PROGRAM p10_directionalInterlock
VAR
	interlockS0: TOF;
	interlockS1: TOF;
	S0: BOOL;	
	S1: BOOL;
	L0: BOOL;
	L1: BOOL;
END_VAR

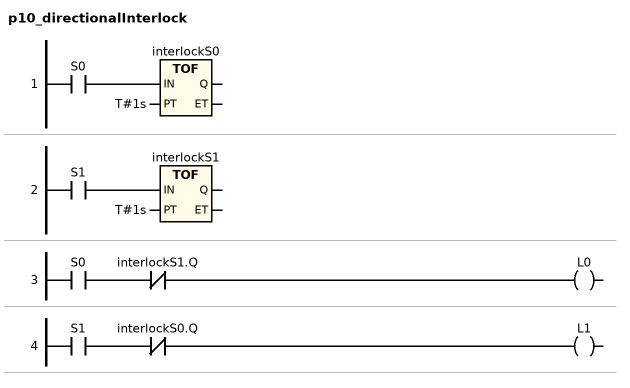
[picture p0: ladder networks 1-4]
// NETWORK 1
interlockS0(IN := S0, PT := T#1s); // TOF

// NETWORK 2
interlockS1(IN := S1, PT := T#1s); // TOF

// NETWORK 3
L0 := S0 AND NOT interlockS1.Q;

// NETWORK 4
L1 := S1 AND NOT interlockS0.Q;

END_PROGRAM
